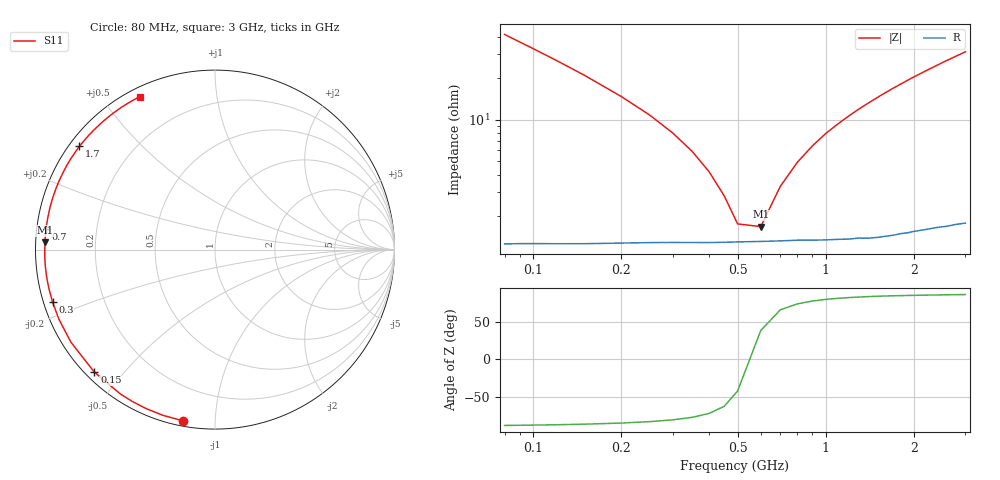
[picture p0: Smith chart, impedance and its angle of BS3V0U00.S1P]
! SIEMENS Small Signal Semiconductors
! BB640
! Si Tuning Diode in SOD323
! VR = 3 V
! S-Parameters:  July  1993
# GHz  S  MA  R  50
!  f  S11
! GHz  MAG  ANG
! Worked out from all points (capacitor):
!   33 points, 80 MHz to 3 GHz, reference 50 ohm
!   read as one part to ground: C = 46.9 pF near 80 MHz
!   lowest |Z| = 1.67 ohm at 600 MHz (marker M1)
!   series resonance near 552.9 MHz, so ESL is about 1.8 nH
!   S11 on the Smith chart (normalised r, x): 80 MHz: 0.03, -0.83; 150 MHz: 0.03, -0.42; 300 MHz: 0.03, -0.16; 700 MHz: 0.03, +0.06; 1.7 GHz: 0.03, +0.34; 3 GHz: 0.04, +0.62
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0.08  0.9708 -100.5
0.09  0.9678 -107.4
0.1  0.9654 -113.4
0.11  0.9634 -118.7
0.12  0.9618 -123.3
0.15  0.9581 -134.5
0.2  0.9543 -147.2
0.25  0.9522 -155.7
0.3  0.9511 -162.0
0.35  0.9506 -166.9
0.4  0.9503 -170.9
0.45  0.9499 -174.3
0.5  0.9495 -177.3
0.6  0.9491 177.6
0.7  0.9488 173.1
0.8  0.9485 169.2
0.9  0.9488 165.6
1  0.949 162.2
1.2  0.9493 156.1
1.4  0.9497 150.5
1.6  0.9494 145.2
1.7  0.9493 142.7
2  0.9484 135.6
2.2  0.9484 131.3
2.4  0.9484 127.2
2.6  0.9491 123.3
2.8  0.9493 119.7
3  0.9501 116.2
